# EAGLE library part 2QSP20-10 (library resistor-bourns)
BOURNS RESISTOR NETWORK
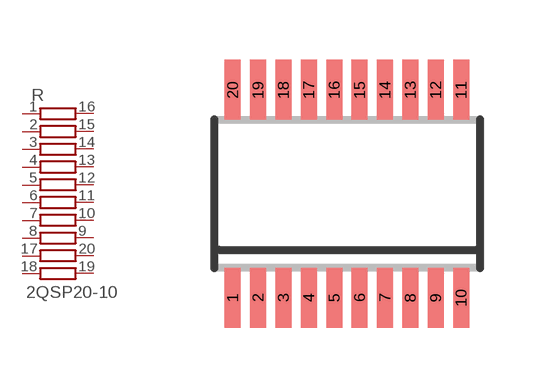
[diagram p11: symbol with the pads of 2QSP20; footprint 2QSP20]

Designator prefix R

## 2QSP20-10 (MF: BOURNS, INC.; MPN: 2QSP20-RG1-100; OC_FARNELL: unknown; OC_NEWARK: 61H1407)  [2QSP20]
1  1  pas
2  2  pas
3  3  pas
4  4  pas
5  5  pas
6  6  pas
7  7  pas
8  8  pas
9  9  pas
10  10  pas
11  11  pas
12  12  pas
13  13  pas
14  14  pas
15  15  pas
16  16  pas
17  17  pas
18  18  pas
19  31  pas
20  32  pas

## Footprint 2QSP20 (pad centres in mm)
BOURNS RESISTOR NETWORK
smd 0.4 x 1.5: 1 -2.223,-2.6; 2 -1.588,-2.6; 3 -0.953,-2.6; 4 -0.318,-2.6; 5 0.318,-2.6; 6 0.953,-2.6; 7 1.588,-2.6; 8 2.223,-2.6; 9 2.858,-2.6; 10 3.493,-2.6; 11 3.493,2.6; 12 2.858,2.6; 13 2.223,2.6; 14 1.588,2.6; 15 0.953,2.6; 16 0.318,2.6; 17 -0.318,2.6; 18 -0.953,2.6; 19 -1.588,2.6; 20 -2.223,2.6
